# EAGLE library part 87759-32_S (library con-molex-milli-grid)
HEADER
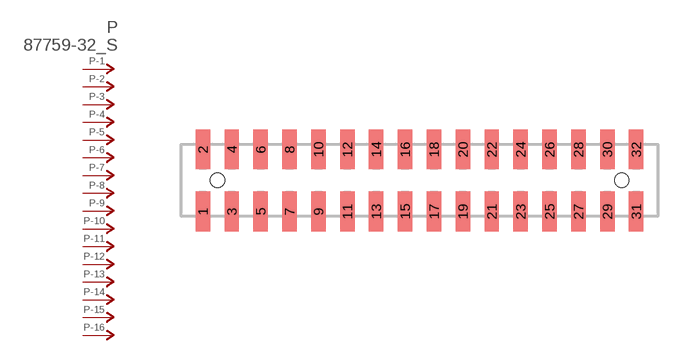
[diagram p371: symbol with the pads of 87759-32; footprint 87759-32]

Designator prefix P; gates -1=P-NV -2=P-N -3=P-N -4=P-N -5=P-N -6=P-N -7=P-N -8=P-N -9=P-N -10=P-N -11=P-N -12=P-N -13=P-N -14=P-N -15=P-N -16=P-N -17=P-N -18=P-N -19=P-N -20=P-N -21=P-N -22=P-N -23=P-N -24=P-N -25=P-N -26=P-N -27=P-N -28=P-N -29=P-N -30=P-N -31=P-N -32=P-N

## 87759-32_S  [87759-32]
1  -1:P  pas
2  -2:P  pas
3  -3:P  pas
4  -4:P  pas
5  -5:P  pas
6  -6:P  pas
7  -7:P  pas
8  -8:P  pas
9  -9:P  pas
10  -10:P  pas
11  -11:P  pas
12  -12:P  pas
13  -13:P  pas
14  -14:P  pas
15  -15:P  pas
16  -16:P  pas
17  -17:P  pas
18  -18:P  pas
19  -19:P  pas
20  -20:P  pas
21  -21:P  pas
22  -22:P  pas
23  -23:P  pas
24  -24:P  pas
25  -25:P  pas
26  -26:P  pas
27  -27:P  pas
28  -28:P  pas
29  -29:P  pas
30  -30:P  pas
31  -31:P  pas
32  -32:P  pas

## Footprint 87759-32 (pad centres in mm)
HEADER SMD Dual Row, Vertical
smd 1 x 2.75: 1 -15,-2.15; 2 -15,2.15; 3 -13,-2.15; 4 -13,2.15; 5 -11,-2.15; 6 -11,2.15; 7 -9,-2.15; 8 -9,2.15; 9 -7,-2.15; 10 -7,2.15; 11 -5,-2.15; 12 -5,2.15; 13 -3,-2.15; 14 -3,2.15; 15 -1,-2.15; 16 -1,2.15; 17 1,-2.15; 18 1,2.15; 19 3,-2.15; 20 3,2.15; 21 5,-2.15; 22 5,2.15; 23 7,-2.15; 24 7,2.15; 25 9,-2.15; 26 9,2.15; 27 11,-2.15; 28 11,2.15; 29 13,-2.15; 30 13,2.15; 31 15,-2.15; 32 15,2.15
hole 1 at -14,0
hole 1 at 14,0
